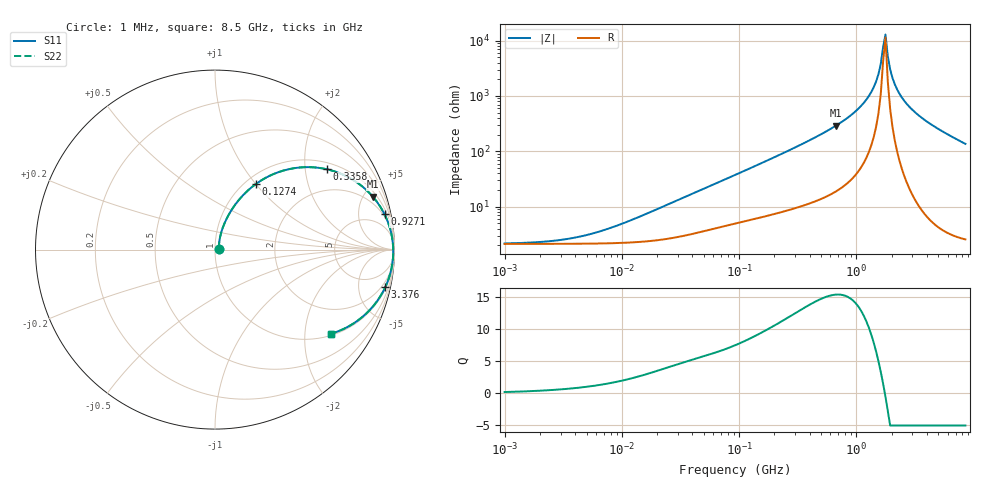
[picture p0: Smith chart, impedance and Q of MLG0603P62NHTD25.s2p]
! S-Parameter Data Generated by TDK Corporation
! Copyright(C) 2025 TDK Corporation.
! All Rights Reserved.
! TDK P/N: MLG0603P62NHTD25 (SMD / SMT Inductor (Coil))
! Property: L=62nH at 300MHz
! Size(LxWxT): 0.6x0.3x0.3mm
! Model Type: s2p (Touchstone File Format Version 1.0)
! Frequency: DC=Yes Start=1MHz Stop=8500MHz 198points Log-sweep
! Model Generated on Feb. 6, 2025
! Terms and conditions regarding TDK Simulation Models:
! 1)This simulation model is being provided solely for informational
!  purposes. Please refer to the specifications of the products in
!  terms of detailed characteristics of such products.
! 2)In no event shall TDK Corporation of any of its subsidiaries be
!  liable for any loss or damage arising, directly or indirectly,
!  from any information contained in this simulation model, including,
!  but not limited to loss or damages arising from any inaccuracies,
!  omissions or errors in connection with such information.
! 3)Any and all copyrights on this simulation model are owned by
!  TDK Corporation.  Duplication or redistribution of this simulation
!  model without prior written permission from TDK Corporation
!  is prohibited.
! 4)This simulation model is subject to any modification or change
!  without any prior notice.
! 5)Neither TDK Corporation nor any of its subsidiaries shall make any
!  warranty, express or implied, including but not limited to the
!  correctness, implied warranties of merchantability and fitness for
!  a particular purpose with respect to this simulation models.
! 6)The use of this simulation model shall be deemed to have consented
!  to the terms and conditions hereof.
! Port Assignments:
!  1 ---@@@--- 2
! Applicable Conditions:
!  Temperature = 25 degC
!  DC Bias Current = 0 A
!  Small Signal Operation
# Hz S MA R 50
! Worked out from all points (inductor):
!   197 points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, 1 MHz to 8.5 GHz, reference 50 ohm
!   read as one part in series: L = 68.9 nH near 16.71 MHz
!   highest Q = 15.4 at 671.1 MHz (marker M1), where L = 68.9 nH
!   self-resonance near 1.689 GHz
!   S11 on the Smith chart (normalised r, x): 1 MHz: 1.04, +0.01; 127.4 MHz: 1.12, +1.01; 335.8 MHz: 1.20, +2.63; 927.1 MHz: 1.65, +9.45; 3.376 GHz: 1.21, -9.00; 8.5 GHz: 1.05, -2.72
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1000000  0.02121 11.4  0.9792 -0.2  0.9792 -0.2  0.02121 11.4
4587603  0.02875 42.1  0.9789 -1.1  0.9789 -1.1  0.02875 42.1
2.10461e7  0.09178 69.5  0.9717 -5.1  0.9717 -5.1  0.09178 69.5
9.219544e7  0.3352 63.0  0.8988 -19.4  0.8988 -19.4  0.3352 63.0
1.273638e8  0.4319 58.0  0.8537 -25.4  0.8537 -25.4  0.4319 58.0
2.216269e8  0.6269 46.2  0.7246 -38.6  0.7246 -38.6  0.6269 46.2
3.357802e8  0.7686 35.6  0.5836 -50.0  0.5836 -50.0  0.7686 35.6
4.229561e8  0.8342 29.6  0.4954 -56.3  0.4954 -56.3  0.8342 29.6
6.710824e8  0.9275 18.5  0.3185 -67.8  0.3185 -67.8  0.9275 18.5
9.270694e8  0.9651 11.7  0.2038 -74.3  0.2038 -74.3  0.9651 11.7
1.222927e9  0.9836 6.4  0.1126 -78.4  0.1126 -78.4  0.9836 6.4
1.470933e9  0.9903 3.1  0.05458 -78.2  0.05458 -78.2  0.9903 3.1
1.613203e9  0.9922 1.4  0.0263 -72.0  0.0263 -72.0  0.9922 1.4
1.689417e9  0.9928 0.6  0.01302 -55.9  0.01302 -55.9  0.9928 0.6
1.769233e9  0.9931 -0.2  0.007706 26.8  0.007706 26.8  0.9931 -0.2
1.852819e9  0.9932 -1.0  0.01905 68.7  0.01905 68.7  0.9932 -1.0
1.940355e9  0.9931 -1.9  0.03292 77.0  0.03292 77.0  0.9931 -1.9
2.128028e9  0.9922 -3.5  0.06167 81.0  0.06167 81.0  0.9922 -3.5
2.333852e9  0.9903 -5.2  0.09105 81.3  0.09105 81.3  0.9903 -5.2
3.37643e9  0.9714 -12.5  0.2159 76.2  0.2159 76.2  0.9714 -12.5
5.115526e9  0.9209 -22.0  0.3748 67.0  0.3748 67.0  0.9209 -22.0
8.5e9  0.799 -35.9  0.5865 53.0  0.5865 53.0  0.799 -35.9
